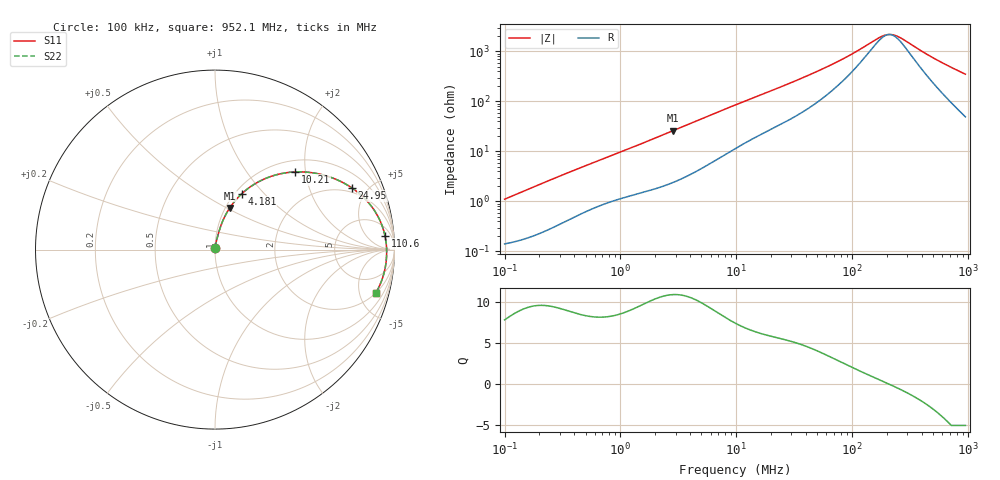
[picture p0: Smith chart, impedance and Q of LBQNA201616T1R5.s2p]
! LBQNA201616T1R5  S-PARAMETER MODEL  ( General Type )
! Model Generated by TAIYO YUDEN Corporation (http://www.ty-top.com)
! Version 1.0
! TAIYO YUDEN Control No. 191025NI43SB-FBB
! Copyright(c) 2019 TAIYO YUDEN CO.,LTD. All Rights Reserved.
! Product Description (link to TY-COMPAS)
! https://ds.yuden.co.jp/TYCOMPAS/or/detail?pn=LBQNA201616T1R5M&u=M
! Products Name : Inductors
! Characteristics :
!  Inductance : 1.5 uH , SRF(min) : 80 MHz , DC Resistance(max) : 0.143 Ohm
!  Rated Current : Saturation :550 mA , Temp Rise : 650 mA (20 degC)
!  Case Size : 2.0 x 1.6 / 0.079 x 0.063 [mm/inch] , Thickness : 1.6 / 0.063 [mm/inch]
!  (Conditions: Temperature = 25 degC , DC Bias Current/Voltage = 0A / 0V)
! External Node Assignments :
!  1  o---GGG---o  2
! GND o---------o GND
! Frequency Range : 0.1MHz  -  952.093921MHz  [ 402 STEP ]
# MHz S RI R 50
! Freq[MHz].  S11 Real  S11 Imag  S21 Real  S21 Imag  S12 Real  S12 Imag  S22 Real  S22 Imag
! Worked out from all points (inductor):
!   401 points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, 100 kHz to 952.1 MHz, reference 50 ohm
!   read as one part in series: L = 1.75 uH near 104.7 kHz
!   highest Q = 10.8 at 2.833 MHz (marker M1), where L = 1.45 uH
!   self-resonance near 209 MHz
!   S11 on the Smith chart (normalised r, x): 100 kHz: 1.00, +0.02; 4.181 MHz: 1.07, +0.75; 10.21 MHz: 1.24, +1.75; 24.95 MHz: 1.72, +3.95; 110.6 MHz: 11, +18; 952.1 MHz: 1.99, -6.95
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0.1  0.00153 0.011  0.9985 -0.011  0.9985 -0.011  0.00153 0.011
0.463905  0.00798 0.0475  0.992 -0.0475  0.992 -0.0475  0.00798 0.0475
1.082572  0.0221 0.1003  0.9779 -0.1003  0.9779 -0.1003  0.0221 0.1003
2.152077  0.0544 0.1841  0.9456 -0.1841  0.9456 -0.1841  0.0544 0.1841
2.832814  0.0819 0.232  0.9181 -0.232  0.9181 -0.232  0.0819 0.232
4.181307  0.1478 0.31  0.8522 -0.31  0.8522 -0.31  0.1478 0.31
6.171716  0.2553 0.3844  0.7447 -0.3844  0.7447 -0.3844  0.2553 0.3844
9.983587  0.4363 0.4323  0.5637 -0.4323  0.5637 -0.4323  0.4363 0.4323
10.21488  0.4456 0.4328  0.5544 -0.4328  0.5544 -0.4328  0.4456 0.4328
15.42673  0.6074 0.4146  0.3926 -0.4146  0.3926 -0.4146  0.6074 0.4146
24.95483  0.7635 0.3431  0.2365 -0.3431  0.2365 -0.3431  0.7635 0.3431
45.26565  0.8837 0.2246  0.1163 -0.2246  0.1163 -0.2246  0.8837 0.2246
73.22333  0.9293 0.1375  0.0707 -0.1375  0.0707 -0.1375  0.9293 0.1375
110.5834  0.9471 0.0769  0.0529 -0.0769  0.0529 -0.0769  0.9471 0.0769
170.8745  0.9549 0.0233  0.0451 -0.0233  0.0451 -0.0233  0.9549 0.0233
191.6068  0.9558 0.01  0.0442 -0.01  0.0442 -0.01  0.9558 0.01
209.9895  0.9563 -0.000575  0.0437 0.000575  0.0437 0.000575  0.9563 -0.000575
230.1359  0.9565 -0.0112  0.0435 0.0112  0.0435 0.0112  0.9565 -0.0112
258.0584  0.9564 -0.0247  0.0436 0.0247  0.0436 0.0247  0.9564 -0.0247
513.0018  0.9445 -0.1194  0.0555 0.1194  0.0555 0.1194  0.9445 -0.1194
723.3016  0.9247 -0.1826  0.0753 0.1826  0.0753 0.1826  0.9247 -0.1826
952.0939  0.8955 -0.2431  0.1045 0.2431  0.1045 0.2431  0.8955 -0.2431
